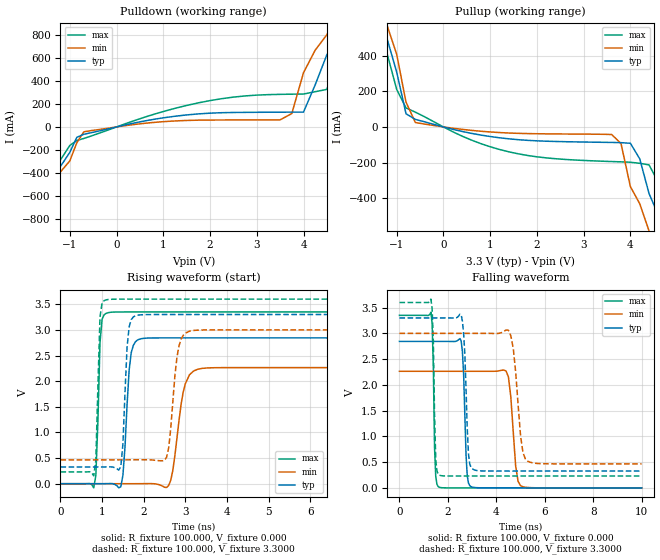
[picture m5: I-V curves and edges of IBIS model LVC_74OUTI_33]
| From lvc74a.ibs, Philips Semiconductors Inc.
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|   Model LVC_74OUTI_33
[Model]   LVC_74OUTI_33
Model_type   Output
Polarity   Inverting
Vmeas =  1.5000V
Cref  = 50.0000pF
Rref  =  0.5000k
Vref  =  0.000V
C_comp   3.12pF   2.70pF   3.60pF
[Model Spec]
| Note: The input and output voltage ratings may be exceeded if the input and
|   output current ratings are observed (please refer to the data sheet)
|   Subparameter   typ   min   max
| Timing Thresholds
Vmeas   1.5   1.5   1.5
|Ambient temperature:   25.0000   85.0000   -40.0000
[Temperature Range]   40.0000   100.0000   -25.0000
[Voltage Range]   3.3000V   3.0000V   3.6000V
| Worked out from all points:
|   slope of the pulldown table from 0 to 0.495 V, typ, clamps not added: 11.4 ohm
|   slope of the pullup table from 0 to 0.495 V, typ, clamps not added: 16.3 ohm
|   rising waveform, R_fixture 100.000, V_fixture 0.000: 20-80 % time 122ps typ, 224ps min, 73.5ps max; typ from 0 V to 2.84 V
|   rising waveform, R_fixture 100.000, V_fixture 3.3000: 20-80 % time 97.8ps typ, 168ps min, 72.3ps max; typ from 0.327 V to 3.3 V
|   falling waveform, R_fixture 100.000, V_fixture 0.000: 20-80 % time 116ps typ, 207ps min, 79.5ps max; typ from 2.84 V to 0 V
|   falling waveform, R_fixture 100.000, V_fixture 3.3000: 20-80 % time 137ps typ, 267ps min, 86.9ps max; typ from 3.3 V to 0.327 V
|Process Range   nominal   slow   fast
[Pulldown]
| voltage   I(typ)   I(min)   I(max)
-5.5V     -4.565A    -4.587A    -4.56A
-1.9V     -966.9mA   -1.009A    -918.8mA
-1.75V    -820.5mA   -863.1mA   -771mA
-1.3V     -396.9mA   -441.3mA   -346.4mA
-700mV    -63.6mA    -42.24mA   -99.98mA
3.5V      127.9mA    61.26mA    282.4mA
3.75V     128.1mA    116.3mA    283.9mA
4V        128.6mA    470mA      285mA
4.5V      626.1mA    799.2mA    325.5mA
4.75V     782.1mA    1.022A     640.2mA
5.25V     1.248A     1.521A     1.043A
11V       6.813A     7.149A     6.482A
[Pullup]
| voltage   I(typ)   I(min)   I(max)
-8V       7.128A     7.158A     7.111A
-1.6V     745.1mA    798.2mA    688.7mA
-1.2V     489.8mA    565.9mA    406.9mA
-800mV    73.9mA     139.3mA    106.8mA
-600mV    42.4mA     24.62mA    82.8mA
1.2V      -60.89mA   -31.54mA   -126.5mA
3.6V      -87.04mA   -42.47mA   -194.3mA
3.8V      -88.38mA   -93.57mA   -196mA
4V        -91.76mA   -334.9mA   -198.2mA
4.4V      -374.8mA   -584.4mA   -213.2mA
5V        -890.2mA   -1.178A    -648.8mA
9.1V      -5.158A    -5.385A    -5.025A
[Ramp]
| variable   typ   min   max
dV/dt_r   1.706V/121.822ps   1.359V/224.056ps   2.010V/73.473ps
dV/dt_f   1.784V/137.324ps   1.521V/266.558ps   2.022V/86.926ps
R_load = 100.000
[Rising Waveform]
R_fixture   = 100.000
V_fixture   = 0.000
V_fixture_min = 0.000
V_fixture_max = 0.000
| time   V(typ)   V(min)   V(max)
0s        116.3pV    3.037nV    937.7pV
800ps     -40.85uV   4.954uV    -81.09mV
950ps     -102.5uV   -6.457uV   2.752V
1.1ns     657.9uV    -12.32uV   3.324V
1.45ns    -61.02mV   -28.48uV   3.349V
1.7ns     2.555V     -107.7uV   3.35V
1.9ns     2.819V     302.3uV    3.35V
2.6ns     2.844V     -33.78mV   3.35V
3.3ns     2.844V     2.233V     3.35V
10ns      2.844V     2.264V     3.35V
[Rising Waveform]
R_fixture   = 100.000
V_fixture   = 3.3000
V_fixture_min = 3.0000
V_fixture_max = 3.6000
| time   V(typ)   V(min)   V(max)
0s        326.6mV    465.6mV    230.2mV
800ps     326.6mV    465.6mV    153.2mV
950ps     326.5mV    465.6mV    3.25V
1.05ns    326.8mV    465.6mV    3.571V
1.45ns    334.4mV    465.7mV    3.6V
1.6ns     2.661V     465.7mV    3.6V
1.8ns     3.275V     465.9mV    3.6V
2.55ns    3.3V       518mV      3.6V
3.1ns     3.3V       2.975V     3.6V
10ns      3.3V       3V         3.6V
[Falling Waveform]
R_fixture   = 100.000
V_fixture   = 0.000
V_fixture_min = 0.000
V_fixture_max = 0.000
| time   V(typ)   V(min)   V(max)
0s        2.844V     2.264V     3.35V
1.3ns     2.844V     2.264V     3.411V
1.45ns    2.844V     2.264V     771.9mV
1.6ns     2.844V     2.264V     23.68mV
2.55ns    2.848V     2.264V     196.4nV
2.8ns     234.5mV    2.264V     13.96nV
2.95ns    24.91mV    2.264V     7.081nV
4.4ns     866.6nV    2.27V      1.519nV
5ns       14.77nV    43.65mV    1.549nV
10ns      150.4pV    4.487nV    1.479nV
[Falling Waveform]
R_fixture   = 100.000
V_fixture   = 3.3000
V_fixture_min = 3.0000
V_fixture_max = 3.6000
| time   V(typ)   V(min)   V(max)
0s        3.3V       3V         3.6V
1.3ns     3.3V       3V         3.665V
1.4ns     3.3V       3V         2.826V
1.5ns     3.3V       3V         538.5mV
1.65ns    3.3V       3V         247.1mV
2.55ns    3.36V      3V         230.2mV
3ns       372.7mV    3V         230.2mV
4.6ns     326.6mV    2.953V     230.2mV
5.3ns     326.6mV    517mV      230.2mV
10ns      326.6mV    465.6mV    230.2mV
